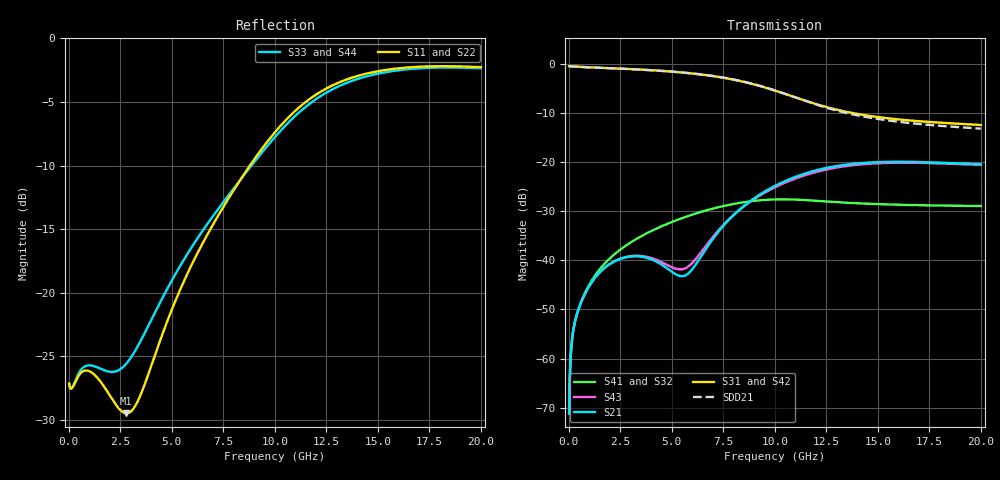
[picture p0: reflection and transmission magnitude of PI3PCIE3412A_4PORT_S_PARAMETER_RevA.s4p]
! NPort=4 DATA=800 NOISE=0 GROUPDELAY=0 COMPLEX_DATAFORMAT=POLAR
! NumOfBlock=1 NumOfParam=0
! .MODEL Smodel S TSTONEFILE=PI3PCIE3412A_4PORT_S_PARAMETER_RevA.s4p TYPE=S
!  -- The above .MODEL line can be used for the S element in the netlist.
!PORT1 = INPUT+
!PORT2 = INPUT-
!PORT3 = OUTPUT+
!PORT4 = OUTPUT-
# Hz S MA R  50
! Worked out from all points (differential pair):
!   800 points, 25 MHz to 20 GHz, reference 50 ohm
!   strongest paths, dB at 25 MHz, 5.025 GHz, 10.03 GHz, 15.03 GHz, 20 GHz:
!     S31: -0.4, -1.5, -5.4, -10.8, -12.4
!     S42: -0.4, -1.6, -5.4, -10.8, -12.4
!     S21: -71.1, -42.4, -24.8, -20.0, -20.4
!     S43: -71.1, -41.4, -25.1, -20.2, -20.5
!     S41: -71.2, -32.2, -27.6, -28.5, -28.9
!     S32: -71.2, -32.2, -27.6, -28.5, -28.9
!   taken as a pair (ports 1,2 in; 3,4 out), SDD21 dB: -0.4, -1.5, -5.4, -11.2, -13.2
!   lowest |S11| = -29.5 dB at 2.8 GHz (marker M1), VSWR 1.07, Z = 53.4 + j0.754 ohm
!   |S11| at or under -10 dB: start of sweep to 8.793 GHz
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2.5e7  0.04403 -2.3  0.0002773 86.0  0.9516 -0.6  0.0002768 86.0
       0.0002773 86.0  0.04403 -2.3  0.0002768 86.0  0.9516 -0.6
       0.9516 -0.6  0.0002768 86.0  0.04402 -2.1  0.0002773 86.0
       0.0002768 86.0  0.9516 -0.6  0.0002773 86.0  0.04402 -2.1
6.5e8  0.0489 2.5  0.003932 64.6  0.9333 -10.2  0.003983 63.8
       0.003932 64.6  0.04887 2.4  0.003983 63.8  0.9333 -10.2
       0.9333 -10.2  0.003983 63.8  0.0504 7.9  0.00393 64.8
       0.003983 63.8  0.9333 -10.2  0.00393 64.8  0.05037 7.8
2.8e9  0.03362 12.1  0.01077 50.5  0.893 -41.0  0.01425 45.2
       0.01078 50.5  0.03339 12.1  0.01425 45.2  0.8929 -41.0
       0.8932 -40.9  0.01425 45.2  0.05268 22.0  0.01085 52.1
       0.01425 45.2  0.893 -40.9  0.01085 52.1  0.05249 22.0
5.675e9  0.1148 44.0  0.007052 85.6  0.8138 -82.9  0.02774 8.9
         0.007051 85.6  0.1148 44.2  0.02774 8.9  0.8136 -82.9
         0.814 -82.8  0.02774 9.0  0.1385 30.0  0.008345 84.4
         0.02774 9.0  0.8138 -82.8  0.008345 84.4  0.1384 30.1
9.175e9  0.3498 14.3  0.04536 108.8  0.606 -135.9  0.04073 -44.2
         0.04536 108.8  0.35 14.4  0.04073 -44.2  0.6057 -135.9
         0.6062 -135.8  0.04075 -44.2  0.3398 6.2  0.04448 104.8
         0.04075 -44.2  0.6059 -135.8  0.04447 104.8  0.3399 6.3
1.2975e10  0.6637 -32.2  0.09131 66.0  0.3443 -174.7  0.03921 -98.4
           0.0913 66.0  0.6639 -32.2  0.03922 -98.4  0.344 -174.6
           0.3445 -174.5  0.03924 -98.3  0.6415 -34.0  0.08814 65.2
           0.03924 -98.3  0.3442 -174.5  0.08814 65.2  0.6418 -34.0
2e10  0.7712 -83.7  0.09536 18.9  0.2391 127.5  0.03577 -179.7
      0.09536 19.0  0.7714 -83.7  0.03577 -179.7  0.2391 127.5
      0.2394 127.7  0.03581 -179.5  0.7636 -84.1  0.09409 19.2
      0.03581 -179.5  0.2393 127.7  0.09409 19.2  0.7637 -84.1
